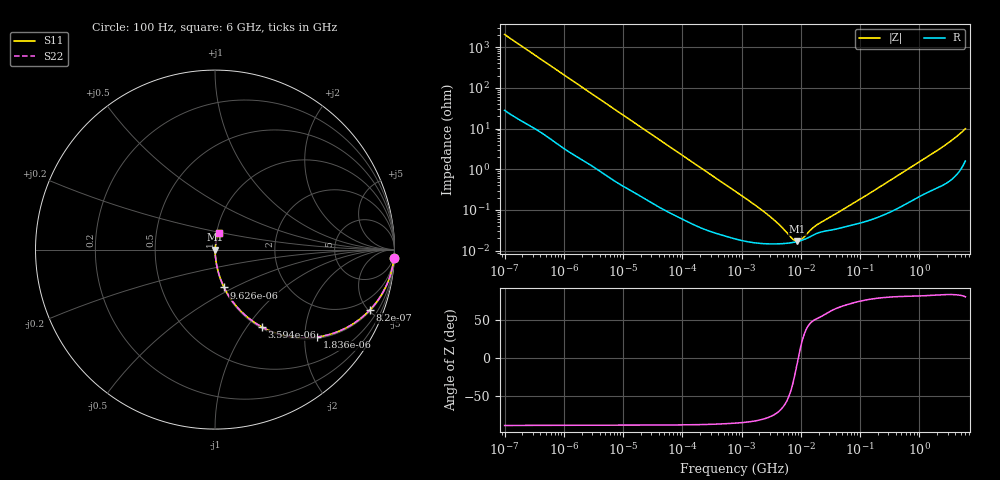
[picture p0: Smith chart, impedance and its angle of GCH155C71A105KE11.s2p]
!Murata Part Number: GCH155C71A105KE11
!These Parameters are Measured in Series Mode Connection
!Data Generated on Jun 19, 2026
!  o--ll--o
!Port1  Port2
!  o------o
!Operation Temp=25[degC], DC Bias Voltage=0[V]
!Freq. Start=100[Hz] Stop=6[GHz] 401[Steps]
# Hz S RI R 50
!Freq.(Hz) S11(Real) S11(Imag) S21(Real) S21(Imag) S12(Real) S12(Imag) S22(Real) S22(Imag)
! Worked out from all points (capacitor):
!   401 points, 100 Hz to 6 GHz, reference 50 ohm
!   read as one part in series: C = 774 nF near 109 Hz
!   lowest |Z| = 16.8 mohm at 8.692 MHz (marker M1)
!   series resonance near 9.062 MHz, so ESL is about 400 pH
!   S11 on the Smith chart (normalised r, x): 100 Hz: 2, -41; 820 Hz: 1.08, -5.10; 1.836 kHz: 1.04, -2.30; 3.594 kHz: 1.02, -1.18; 9.626 kHz: 1.01, -0.45; 6 GHz: 1.03, +0.20
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100  0.997 -0.0486  0.00304 0.0486  0.00304 0.0486  0.997 -0.0486
293  0.9783 -0.1382  0.0217 0.1382  0.0217 0.1382  0.9783 -0.1382
524  0.9371 -0.2349  0.0629 0.2349  0.0629 0.2349  0.9371 -0.2349
820  0.863 -0.3362  0.137 0.3362  0.137 0.3362  0.863 -0.3362
1174  0.7584 -0.4204  0.2416 0.4204  0.2416 0.4204  0.7584 -0.4204
1836  0.5674 -0.4874  0.4326 0.4874  0.4326 0.4874  0.5674 -0.4874
2008  0.5242 -0.4913  0.4758 0.4913  0.4758 0.4913  0.5242 -0.4913
3594  0.2623 -0.4314  0.7377 0.4314  0.7377 0.4314  0.2623 -0.4314
5625  0.13 -0.3279  0.87 0.3279  0.87 0.3279  0.13 -0.3279
9626  0.0507 -0.2107  0.9493 0.2107  0.9493 0.2107  0.0507 -0.2107
18841  0.0152 -0.1127  0.9848 0.1127  0.9848 0.1127  0.0152 -0.1127
40335  0.00408 -0.0538  0.9959 0.0538  0.9959 0.0538  0.00408 -0.0538
774597  0.000203 -0.00291  0.9998 0.00291  0.9998 0.00291  0.000203 -0.00291
2837864  0.000148 -0.00073  0.9999 0.00073  0.9999 0.00073  0.000148 -0.00073
4440638  0.000148 -0.000392  0.9999 0.000392  0.9999 0.000392  0.000148 -0.000392
7266822  0.000159 -0.000112  0.9998 0.000112  0.9998 0.000112  0.000159 -0.000112
8692127  0.000167 -2.07e-05  0.9998 2.07e-05  0.9998 2.07e-05  0.000167 -2.07e-05
1.039699e7  0.00018 6.82e-05  0.9998 -6.82e-05  0.9998 -6.82e-05  0.00018 6.82e-05
1.555665e7  0.000234 0.000262  0.9998 -0.000262  0.9998 -0.000262  0.000234 0.000262
3.124326e8  0.000893 0.0051  0.9991 -0.0051  0.9991 -0.0051  0.000893 0.0051
2.240541e9  0.00473 0.0317  0.9953 -0.0317  0.9953 -0.0317  0.00473 0.0317
6e9  0.0248 0.0942  0.9752 -0.0942  0.9752 -0.0942  0.0248 0.0942
